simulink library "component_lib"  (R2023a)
settings: Solver=VariableStepAuto  StartTime=0.0  StopTime=10.0  RelTol=1e-3
undefined symbols (not defined in the file or in its folder): component_lib, ECCV_r, KoblenzTrier, mm, par, param_TD04, R1234yf_ph, SigIdentifier, Systems, TH0023_WP120, Thermal, V_nom
libraries: base_lib x166, $bdroot x164, simulink x2, slpidlib x1
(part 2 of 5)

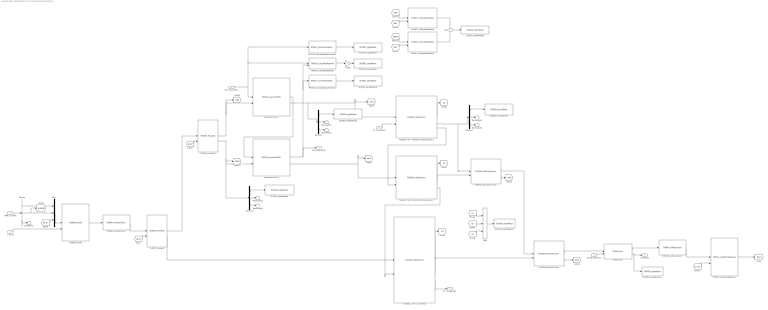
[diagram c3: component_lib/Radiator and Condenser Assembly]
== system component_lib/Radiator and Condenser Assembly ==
  AMB: (T,p,RH) : Inport
  v [m/s] : Inport  Port=2
  rel_fan_speed [-] : Inport  Port=3
  CL: (T1,p1,W1) : Inport  Port=4
  RF: (h1,p1,W1) : Inport  Port=5
  Add : Sum  Inputs=+++
  Condenser Pass 1 : $bdroot/Thermal Systems/RF0012_louverFinHEX  N_tub=40  T_L=0.95  T_p=10.15e-3  T_d=16e-3  N_ch=18  a=1.3e-3  b=0.58e-3  L_a=23  F_p=1.4e-3  L_p=1.7e-3  L_l=6.4e-3  H=8.15e-3  d_f=16e-3  F_d=16e-3  N_nod=5
  Condenser Pass 2 : $bdroot/Thermal Systems/RF0012_louverFinHEX  N_tub=40  T_L=0.95  T_p=10.15e-3  T_d=16e-3  N_ch=18  a=1.3e-3  b=0.58e-3  L_a=23  F_p=1.4e-3  L_p=1.7e-3  L_l=6.4e-3  H=8.15e-3  d_f=16e-3  F_d=16e-3  N_nod=5
  Demux{,1..3} (4 alike) : Demux  Outputs=3
  Gain2 : Gain  Gain=-1
  Mux : Mux  Inputs=3
  RF0013_calculateHeatflow : $bdroot/Thermal Systems/RF0013_calculateHeatflow
  RF0014_calculateVaporFraction : $bdroot/Thermal Systems/RF0014_calculateVaporFraction
  RF0014_calculateVaporFraction1 : $bdroot/Thermal Systems/RF0014_calculateVaporFraction
  Radiator core - behind condenser pass 1 : $bdroot/Thermal Systems/TH0002_radiatorCore  HtH=0.4060  StS=0.95  radmodel=52 mm
  Radiator core - behind condenser pass 2 : $bdroot/Thermal Systems/TH0002_radiatorCore  HtH=0.4060  StS=0.95  radmodel=52 mm
  Radiator core - uncovered : $bdroot/Thermal Systems/TH0002_radiatorCore  HtH=1.1- 2 * 0.4060  StS=0.95  radmodel=52 mm
  SC0002_signalRead1 : $bdroot/Data & Control/SC0002_signalRead  SigName=vaporFractionCondenserInlet
  SC0002_signalRead10 : $bdroot/Data & Control/SC0002_signalRead  SigName=vaporFractionCondenserOutlet
  SC0002_signalRead11 : $bdroot/Data & Control/SC0002_signalRead  SigName=fanPower
  SC0002_signalRead12 : $bdroot/Data & Control/SC0002_signalRead  SigName=radiatorCooling
  SC0002_signalRead2 : $bdroot/Data & Control/SC0002_signalRead  SigName=airTemperatureAfterCondenser
  SC0002_signalRead3 : $bdroot/Data & Control/SC0002_signalRead  SigName=airTemperatureAfterRadiator
  SC0002_signalRead4 : $bdroot/Data & Control/SC0002_signalRead  SigName=airTemperatureIntake
  SC0002_signalRead5 : $bdroot/Data & Control/SC0002_signalRead  SigName=condenserAirHeating
  SC0002_signalRead9 : $bdroot/Data & Control/SC0002_signalRead  SigName=condenserCooling
  Sum : Sum  Inputs=+|+
  TH0005_flowSplit : $bdroot/Thermal Systems/TH0005_flowSplit  SystemSampleTime=-1  VariantActivationTime=update diagram  Latency=0  AutoFrameSizeCalculation=off
  TH0005_flowSplit1 : $bdroot/Thermal Systems/TH0005_flowSplit  SystemSampleTime=-1  VariantActivationTime=update diagram  Latency=0  AutoFrameSizeCalculation=off
  TH0006_flowConfluence : $bdroot/Thermal Systems/TH0006_flowConfluence  gain=0.01
  TH0006_flowConfluence1 : $bdroot/Thermal Systems/TH0006_flowConfluence  gain=0.01
  TH0007_airRestriction : $bdroot/Thermal Systems/TH0007_airRestriction  A=0.8  zeta=0.3
  TH0007_airRestriction1 : $bdroot/Thermal Systems/TH0007_airRestriction  A=1  zeta=2.5
  TH0009_intake : $bdroot/Thermal Systems/TH0009_intake  zeta=0.9
  TH0010_fan : $bdroot/Thermal Systems/TH0010_fan  n_fan=4
  TH0011_outletFlowBalance : $bdroot/Thermal Systems/TH0011_outletFlowBalance  gain=0.05
  TH0017_calculateHeatflow : $bdroot/Thermal Systems/TH0017_calculateHeatflow
  TH0017_calculateHeatflow1 : $bdroot/Thermal Systems/TH0017_calculateHeatflow
  Terminator{,1..6} (7 alike) : Terminator
  P_fan [J/s] : Outport
  CL: (T2,p2,W2) : Outport  Port=2
  RF: (h2,p2,W2) : Outport  Port=3
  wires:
  Demux/2 -> Mux/2, [p_amb]
  Demux/1 -> Mux/1
  AMB: (T,p,RH)/1 -> Demux/1
  Radiator core - uncovered/3 -> CL: (T2,p2,W2)/1
  TH0010_fan/2 -> SC0002_signalRead11/1, P_fan [J/s]/1
  rel_fan_speed [-]/1 -> TH0010_fan/2
  v [m/s]/1 -> TH0009_intake/2
  TH0007_airRestriction/1 -> TH0005_flowSplit/1
  TH0007_airRestriction1/1 -> TH0011_outletFlowBalance/1
  TH0006_flowConfluence/1 -> TH0010_fan/1
  Mux/1 -> TH0009_intake/1
  TH0009_intake/1 -> TH0007_airRestriction/1
  Radiator core - uncovered/2 -> TH0006_flowConfluence/2
  [p_amb] -> TH0011_outletFlowBalance/2
  TH0005_flowSplit/2 -> Radiator core - uncovered/1
  TH0010_fan/1 -> TH0007_airRestriction1/1
  TH0011_outletFlowBalance/1 -> [W_in]
  [W_in] -> Mux/3
  Demux/3 -> Terminator/1
  CL: (T1,p1,W1)/1 -> Radiator core - behind condenser pass 1/2
  TH0005_flowSplit/1 -> TH0005_flowSplit1/1
  Condenser Pass 2/1 -> RF0013_calculateHeatflow/2, RF0014_calculateVaporFraction/1, RF: (h2,p2,W2)/1
  Condenser Pass 1/1 -> Condenser Pass 2/1
  Condenser Pass 1/2 -> [AIR1], Radiator core - behind condenser pass 1/1, Demux1/1
  Condenser Pass 2/2 -> [AIR2], Radiator core - behind condenser pass 2/1
  TH0005_flowSplit1/1 -> [AIR0], Condenser Pass 1/2
  Radiator core - behind condenser pass 1/3 -> Radiator core - behind condenser pass 2/2
  Radiator core - behind condenser pass 2/3 -> Radiator core - uncovered/2
  Radiator core - behind condenser pass 2/2 -> TH0006_flowConfluence1/2
  TH0006_flowConfluence1/1 -> TH0006_flowConfluence/1
  [split1] -> TH0005_flowSplit/2
  TH0006_flowConfluence/2 -> [split1]
  [split2] -> TH0005_flowSplit1/2
  TH0006_flowConfluence1/2 -> [split2]
  RF0013_calculateHeatflow/1 -> Gain2/1
  Gain2/1 -> SC0002_signalRead9/1
  Add/1 -> SC0002_signalRead12/1
  RF0014_calculateVaporFraction/1 -> SC0002_signalRead10/1
  RF0014_calculateVaporFraction1/1 -> SC0002_signalRead1/1
  RF: (h1,p1,W1)/1 -> RF0014_calculateVaporFraction1/1, RF0013_calculateHeatflow/1, Condenser Pass 1/1
  Radiator core - behind condenser pass 1/1 -> [Q1]
  Radiator core - behind condenser pass 2/1 -> [Q2]
  Radiator core - uncovered/1 -> [Q3]
  [Q1] -> Add/1
  [Q2] -> Add/2
  [Q3] -> Add/3
  Demux1/2 -> Terminator1/1
  Demux1/3 -> Terminator2/1
  Demux1/1 -> SC0002_signalRead2/1
  Radiator core - behind condenser pass 1/2 -> TH0006_flowConfluence1/1, Demux2/1
  Demux2/3 -> Terminator4/1
  Demux2/2 -> Terminator3/1
  Demux2/1 -> SC0002_signalRead3/1
  TH0005_flowSplit1/2 -> Demux3/1, Condenser Pass 2/2, [AIR00]
  Demux3/3 -> Terminator6/1
  Demux3/2 -> Terminator5/1
  Demux3/1 -> SC0002_signalRead4/1
  [AIR0] -> TH0017_calculateHeatflow/1
  [AIR1] -> TH0017_calculateHeatflow/2
  [AIR2] -> TH0017_calculateHeatflow1/2
  TH0017_calculateHeatflow/1 -> Sum/1
  TH0017_calculateHeatflow1/1 -> Sum/2
  Sum/1 -> SC0002_signalRead5/1
  [AIR00] -> TH0017_calculateHeatflow1/1

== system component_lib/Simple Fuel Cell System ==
  I [A] : Inport
  T [K] : Inport  Port=2
  Constant : Constant  Value=2.5e5
  Constant1 : Constant  Value=0.8
  Constant2 : Constant  Value=2.5e5
  Constant3 : Constant  Value=0.8
  Constant4 : Constant  Value=n
  EL0007_pukrushpan2004 : $bdroot/Electrochemistry/EL0007_pukrushpan2004  U_0=1  j_0=1e-3  alpha=0.25  ASR=1e-1  A_fc=420
  F0010_vaporSaturationPressure.m : base_lib/F0010_gasFlow/F0010_vaporSaturationPressure.m  SystemSampleTime=-1  VariantActivationTime=update diagram  Latency=0  AutoFrameSizeCalculation=off
  GE0002_dynHumidGasSupply : $bdroot/Gas Exchange/GE0002_dynHumidGasSupply  x_H2_dry=0  x_O2_dry=0.21
  GE0002_dynHumidGasSupply1 : $bdroot/Gas Exchange/GE0002_dynHumidGasSupply  x_H2_dry=1  x_O2_dry=0
  Gain : Gain  Gain=n_st
  Gain1 : Gain  Gain=n_st
  Gain2 : Gain  Gain=n_st
  Product{1..5} (5 alike) : Product
  SC0002_signalRead1 : $bdroot/Data & Control/SC0002_signalRead  SigName=fuelCellVoltage
  SC0002_signalRead3 : $bdroot/Data & Control/SC0002_signalRead  SigName=membraneWaterContent
  SC0002_signalRead4 : $bdroot/Data & Control/SC0002_signalRead  SigName=fuelCellPower
  SC0002_signalRead5 : $bdroot/Data & Control/SC0002_signalRead  SigName=vaporSaturationPressure
  SC0002_signalRead6 : $bdroot/Data & Control/SC0002_signalRead  SigName=singleCellVoltage
  SC0002_signalRead8 : $bdroot/Data & Control/SC0002_signalRead  SigName=fuelCellCurrent
  Subsystem1 : Subsystem
  V [V] : Outport
  Q_gen [J/s] : Outport  Port=2
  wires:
  Product1/1 -> Gain1/1
  Product2/1 -> [W_an], Gain/1
  Product5/1 -> [W_ca]
  Constant4/1 -> Product1/2, Product2/2, Product5/2, Product3/2
  EL0007_pukrushpan2004/3 -> Product5/1
  EL0007_pukrushpan2004/2 -> Product2/1
  EL0007_pukrushpan2004/5 -> Product3/1
  Product4/1 -> SC0002_signalRead4/1
  EL0007_pukrushpan2004/4 -> SC0002_signalRead3/1
  T [K]/1 -> F0010_vaporSaturationPressure.m/1, EL0007_pukrushpan2004/4, EL0007_pukrushpan2004/5, EL0007_pukrushpan2004/6, GE0002_dynHumidGasSupply1/1, GE0002_dynHumidGasSupply/1
  F0010_vaporSaturationPressure.m/1 -> SC0002_signalRead5/1
  Gain/1 -> Subsystem1/1(In1)
  Gain1/1 -> V [V]/1, SC0002_signalRead1/1, Product4/2
  Product3/1 -> Gain2/1
  Gain2/1 -> Q_gen [J/s]/1
  GE0002_dynHumidGasSupply1/1 -> EL0007_pukrushpan2004/2
  GE0002_dynHumidGasSupply/1 -> EL0007_pukrushpan2004/3
  I [A]/1 -> EL0007_pukrushpan2004/1, SC0002_signalRead8/1, Product4/1
  EL0007_pukrushpan2004/1 -> SC0002_signalRead6/1, Product1/1
  Constant/1 -> GE0002_dynHumidGasSupply/2
  Constant1/1 -> GE0002_dynHumidGasSupply/3
  Constant3/1 -> GE0002_dynHumidGasSupply1/3
  Constant2/1 -> GE0002_dynHumidGasSupply1/2

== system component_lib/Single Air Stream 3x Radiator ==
  AMB: (T,p,RH) : Inport
  v [m/s] : Inport  Port=2
  rel_fan_speed [-] : Inport  Port=3
  CL A: (T1,p1,W1) : Inport  Port=4
  CL B: (T1,p1,W1) : Inport  Port=5
  CL C: (T1,p1,W1) : Inport  Port=6
  Battery Circuit Radiator : $bdroot/Thermal Systems/TH0002_radiatorCore  HtH=1.1  StS=0.95  radmodel=52 mm
  Demux : Demux  Outputs=3
  Fuel Cell Circuit Radiator : $bdroot/Thermal Systems/TH0002_radiatorCore  HtH=1.1  StS=0.95  radmodel=52 mm
  Fuel Cell Circuit Radiator1 : $bdroot/Thermal Systems/TH0002_radiatorCore  HtH=1.1  StS=0.95  radmodel=52 mm
  Mux : Mux  Inputs=3
  TH0003_coolantTank{,1..5} (6 alike) : $bdroot/Thermal Systems/TH0003_coolantTank  StS=0.95  D_con=0.055  T_0=286  radmodel=52 mm
  TH0004_radiatorPlugFlow : $bdroot/Thermal Systems/TH0004_radiatorPlugFlow  HtH=1.1  StS=0.95  T_0=286  radmodel=52 mm
  TH0004_radiatorPlugFlow1 : $bdroot/Thermal Systems/TH0004_radiatorPlugFlow  HtH=1.1  StS=0.95  T_0=286  radmodel=52 mm
  TH0004_radiatorPlugFlow2 : $bdroot/Thermal Systems/TH0004_radiatorPlugFlow  HtH=1.1  StS=0.95  T_0=286  radmodel=52 mm
  TH0007_airRestriction : $bdroot/Thermal Systems/TH0007_airRestriction  A=0.8  zeta=0.3
  TH0007_airRestriction1 : $bdroot/Thermal Systems/TH0007_airRestriction  A=1  zeta=2.5
  TH0009_intake : $bdroot/Thermal Systems/TH0009_intake  zeta=0.9
  TH0010_fan : $bdroot/Thermal Systems/TH0010_fan  n_fan=10
  TH0011_outletFlowBalance : $bdroot/Thermal Systems/TH0011_outletFlowBalance  gain=0.05
  P_fan [J/s] : Outport
  CL A: (T2,p2,W2) : Outport  Port=2
  CL B: (T2,p2,W2) : Outport  Port=3
  CL C: (T2,p2,W2) : Outport  Port=4
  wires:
  Demux/2 -> Mux/2, [p_amb]
  Demux/1 -> Mux/1
  AMB: (T,p,RH)/1 -> Demux/1
  TH0003_coolantTank1/1 -> CL A: (T2,p2,W2)/1
  TH0010_fan/2 -> P_fan [J/s]/1
  rel_fan_speed [-]/1 -> TH0010_fan/2
  v [m/s]/1 -> TH0009_intake/2
  TH0004_radiatorPlugFlow/1 -> TH0003_coolantTank1/1
  TH0007_airRestriction1/1 -> TH0011_outletFlowBalance/1
  CL A: (T1,p1,W1)/1 -> TH0003_coolantTank/1
  Mux/1 -> TH0009_intake/1
  TH0009_intake/1 -> TH0007_airRestriction/1
  TH0003_coolantTank/1 -> Battery Circuit Radiator/2
  [p_amb] -> TH0011_outletFlowBalance/2
  TH0007_airRestriction/1 -> Battery Circuit Radiator/1
  TH0010_fan/1 -> TH0007_airRestriction1/1
  Battery Circuit Radiator/3 -> TH0004_radiatorPlugFlow/1
  TH0011_outletFlowBalance/1 -> [W_in]
  [W_in] -> Mux/3
  Battery Circuit Radiator/2 -> Fuel Cell Circuit Radiator/1
  Fuel Cell Circuit Radiator/2 -> Fuel Cell Circuit Radiator1/1
  TH0004_radiatorPlugFlow1/1 -> TH0003_coolantTank2/1
  TH0003_coolantTank2/1 -> CL B: (T2,p2,W2)/1
  Fuel Cell Circuit Radiator/3 -> TH0004_radiatorPlugFlow1/1
  Fuel Cell Circuit Radiator1/3 -> TH0004_radiatorPlugFlow2/1
  TH0003_coolantTank3/1 -> CL C: (T2,p2,W2)/1
  TH0004_radiatorPlugFlow2/1 -> TH0003_coolantTank3/1
  TH0003_coolantTank4/1 -> Fuel Cell Circuit Radiator/2
  CL B: (T1,p1,W1)/1 -> TH0003_coolantTank4/1
  TH0003_coolantTank5/1 -> Fuel Cell Circuit Radiator1/2
  CL C: (T1,p1,W1)/1 -> TH0003_coolantTank5/1
  Fuel Cell Circuit Radiator1/2 -> TH0010_fan/1

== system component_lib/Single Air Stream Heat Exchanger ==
  AMB: (T,p,RH) : Inport
  v [m/s] : Inport  Port=2
  rel_fan_speed [-] : Inport  Port=3
  CL: (T1,p1,W1) : Inport  Port=4
  Demux : Demux  Outputs=3
  Mux : Mux  Inputs=3
  Radiator core - exposed : $bdroot/Thermal Systems/TH0002_radiatorCore  HtH=0.6  StS=0.6  radmodel=52 mm
  TH0003_coolantTank : $bdroot/Thermal Systems/TH0003_coolantTank  StS=0.95  D_con=0.055  T_0=286  radmodel=52 mm
  TH0003_coolantTank1 : $bdroot/Thermal Systems/TH0003_coolantTank  StS=0.95  D_con=0.055  T_0=286  radmodel=52 mm
  TH0004_radiatorPlugFlow : $bdroot/Thermal Systems/TH0004_radiatorPlugFlow  HtH=1.1  StS=0.95  T_0=286  radmodel=52 mm
  TH0007_airRestriction : $bdroot/Thermal Systems/TH0007_airRestriction  A=0.8  zeta=0.3
  TH0007_airRestriction1 : $bdroot/Thermal Systems/TH0007_airRestriction  A=1  zeta=2.5
  TH0009_intake : $bdroot/Thermal Systems/TH0009_intake  zeta=0.9
  TH0010_fan : $bdroot/Thermal Systems/TH0010_fan  n_fan=4
  TH0011_outletFlowBalance : $bdroot/Thermal Systems/TH0011_outletFlowBalance  gain=0.05
  P_fan [J/s] : Outport
  CL: (T2,p2,W2) : Outport  Port=2
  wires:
  Demux/2 -> Mux/2, [p_amb]
  Demux/1 -> Mux/1
  AMB: (T,p,RH)/1 -> Demux/1
  TH0003_coolantTank1/1 -> CL: (T2,p2,W2)/1
  TH0010_fan/2 -> P_fan [J/s]/1
  rel_fan_speed [-]/1 -> TH0010_fan/2
  v [m/s]/1 -> TH0009_intake/2
  TH0004_radiatorPlugFlow/1 -> TH0003_coolantTank1/1
  TH0007_airRestriction1/1 -> TH0011_outletFlowBalance/1
  CL: (T1,p1,W1)/1 -> TH0003_coolantTank/1
  Mux/1 -> TH0009_intake/1
  TH0009_intake/1 -> TH0007_airRestriction/1
  TH0003_coolantTank/1 -> Radiator core - exposed/2
  [p_amb] -> TH0011_outletFlowBalance/2
  TH0007_airRestriction/1 -> Radiator core - exposed/1
  TH0010_fan/1 -> TH0007_airRestriction1/1
  Radiator core - exposed/3 -> TH0004_radiatorPlugFlow/1
  TH0011_outletFlowBalance/1 -> [W_in]
  [W_in] -> Mux/3
  Radiator core - exposed/2 -> TH0010_fan/1

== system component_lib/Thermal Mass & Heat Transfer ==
  Q_in [J/s] : Inport
  CL: (T1,p1,W1) : Inport  Port=2
  Sum : Sum  Inputs=|+-
  TH0011_coolingChannel : $bdroot/Thermal Systems/TH0011_coolingChannel  d=d  L=L  n_ch=n
  TH0011_thermalMass : $bdroot/Thermal Systems/TH0011_thermalMass  m=m  cp=cp  T_0=T_0
  T_ [K] : Outport
  CL: (T2,p2,W2) : Outport  Port=2
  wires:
  Sum/1 -> TH0011_thermalMass/1
  TH0011_thermalMass/1 -> T_ [K]/1, TH0011_coolingChannel/1
  TH0011_coolingChannel/1 -> Sum/2
  Q_in [J/s]/1 -> Sum/1
  CL: (T1,p1,W1)/1 -> TH0011_coolingChannel/2
  TH0011_coolingChannel/2 -> CL: (T2,p2,W2)/1

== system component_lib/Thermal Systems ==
  note: TitanX Radiator blockset
  RF0003_compressor : Subsystem  mask{V_disp=0.00017, N_ref=2000}
      mask prompts: V_disp "Displacement Volume [m3]:"; N_ref "Refrence Speed [rpm]:"
      mask init:
      | % fluid properties
      | 
      | par = struct;
      | par.V_disp = V_disp;
      | par.N_ref  = N_ref;
      | 
      | setRefrigerantProperties;
  RF0004_smoothTube : Subsystem  mask{D=8e-3, L=1}
      mask prompts: D "Tube diameter [m]:"; L "Tube length [m]:"
      mask init:
      | % fluid properties
      | 
      | par = struct;
      | par.D = D;
      | par.L = L;
      | 
      | setRefrigerantProperties;
  RF0005_expansionValve : Subsystem  mask{D=1.8e-3, p_min=150e3}
      mask prompts: D "Orifice diameter [m]:"; p_min "Minimum Downstream Pressure [Pa]:"
      mask init:
      | % fluid properties
      | 
      | setRefrigerantProperties;
      | 
      | par.D = D;
  RF0007_PHEX : Subsystem  mask{N_ch=10, L=180e-3, B=65e-3, H=2e-3, t=0.3e-3, D_h=2.61e-3, N_nod=10}
      mask prompts: N_ch "Plates [-]:"; L "Length [m]:"; B "Width [m]:"; H "Height [m]:"; t "Plate thickness [m]"; D_h "Hydraulic Diameter [m]:"; N_nod "Nodes [even integer]"
      mask init:
      | % fluid properties
      | 
      | setRefrigerantProperties;
      | setCoolantProperties;
      | 
      | % Linearly spaced nodes
      | dx = L ./ N_nod;
      | 
      | % flow cross section area
      | A_c = H .* B;
      | 
      | % Volume per node
      | V = B .* H .* dx;
      | 
      | % aluminium properties
      | cp_w     = 0.9e3; % [J/kg K] specific heat
      | k_w      = 237;   % [W / mK] thermal conductivity
      | rho_w    = 2710;
      | A_w      = t .* B;
      | V_w      = t .* B .* dx;
      | d_w      = dx;
      | 
      | % hydraulic diameter
      | par.D_h = D_h;
      | 
      | % heat transfer area for each node
      | A =  2 .* B .* dx;
  RF0008_receiver : Subsystem  mask{V=1e-3, h0=280e3, p0=1e6, p_gain=1e3}
      mask prompts: V "Volume [m3]:"; h0 "Enthalpy [J/kg]:"; p0 "Pressure [Pa]:"; p_gain "Pressure gain:"
      mask init:
      | % fluid properties
      | par = struct;
      | setRefrigerantProperties;
  RF0010_calculateSuperHeat : Subsystem
      mask init:
      | % fluid properties
      | par = struct;
      | setRefrigerantProperties;
  RF0011_calculateSubCool : Subsystem
      mask init:
      | % fluid properties
      | par = struct;
      | setRefrigerantProperties;
  RF0012_louverFinHEX : Subsystem  mask{N_tub=30, T_L=0.3, T_p=10.15e-3, T_d=16e-3, N_ch=18, a=1.3e-3, b=0.58e-3, L_a=23, F_p=1.4e-3, L_p=1.7e-3, L_l=6.4e-3, H=8.15e-3, d_f=16e-3, F_d=16e-3, N_nod=10}
      mask prompts: N_tub "Nr. of Tubes [-]"; T_L "Tube length [m]:"; T_p "Tube pitch [m]:"; T_d "Tube depth [m]:"; N_ch "Minichannels per tube [-]"; a "Minichannel height [m]"; b "Minichannel width [m]"; L_a "Louver angle [deg]:"; F_p "Fin Pitch [m]:"; L_p "Louver Pitch [m]:"; L_l "Louver length [m]:"; H "Fin height [m]:"; d_f "Fin thickness [m]:"; F_d "Flow depth [m]:"; N_nod "Nodes [even integer]"
      mask init:
      | % fluid properties
      | 
      | setRefrigerantProperties;
      | setCoolantProperties;
      | setAirProperties;
      | 
      | % channel parameters
      | par.a = a;
      | par.b = b;
      | 
      | % Louver fin parameters
      | par.L_a  = L_a;  % Louver angle [deg]
      | par.F_p  = F_p;  % Fin pitch [m]
      | par.L_p  = L_p;  % Louver pitch [m]
      | par.L_l  = L_l;  % Louver length [m]
      | par.H    = H;    % Fin height [m]
      | par.T_p  = T_p;  % Tube pitch [m]
      | par.T_d  = T_d;  % Tube depth [m]
      | par.d_f  = d_f;  % Fin thickness [m]
      | par.F_d  = F_d;  % Flow depth [m]
      | 
      | % Aluminium properties
      | cp_w  = 0.9e3; % [J/kg K] specific heat
      | k_w   = 237;   % [W / mK] thermal conductivity
      | rho_w = 2710;
      | 
      | par.cp_w = cp_w;
      | par.k_w = k_w;
      | par.rho_w = rho_w;
      | 
      | 
      | % uniformly spaced nodes
      | dx = T_L ./ N_nod;
      | 
      | % Inner channel surface
      | A_wr = 2.*(a+b) .* dx .*  N_ch;
      | 
      | % Hydraulic diameter
      | D_h =  2 .* a .* b /(a + b);
      | par.D_h = D_h;
      | 
      | % Channel volume per node
      | V = N_ch .* a .* b .* dx;
      | 
      | % approximate number of fins between two tubes
      | n_fin = T_L./F_p;
      | 
      | % Fin surface area per node per tube
      | A_f =  L_l .* F_d .* n_fin ./ N_nod;
      | par.A_f = A_f;
      | 
      | % Tube surfae area per node
      | A_tub = 2 .* dx .* T_d;
      | 
      | % Total surface area per node
      | A_o = A_f + A_tub;
      | par.A_o = A_o;
      | 
      | % free flow cross section area per tube
      | A_fr = T_p .*  T_L;
      | 
      | % minimum cross section area per tube
      | A_min = H .* T_L  - atan( L_a * pi / 180 ) * L_p .* L_l;
      | 
      | % contraction ratio
      | par.sigma = A_fr ./ A_min;
      | 
      | % metal volume per node
      | V_w = (T_d .* (T_p - H)  - a.*b*N_ch ) * dx + A_f .* d_f; 
      | 
      | % node distance
      | d_w = dx;
      | A_w = (T_d .* (T_p - H)  - a.*b*N_ch );
      | 
      | % air volume per node
      | V_air = A_min .* F_d ./ N_nod;
  RF0013_calculateHeatflow : Subsystem
      mask init:
      | % fluid properties
      | par = struct;
      | setRefrigerantProperties;
      | setCoolantProperties;
  RF0014_calculateVaporFraction : Subsystem
      mask init:
      | % fluid properties
      | par = struct;
      | setRefrigerantProperties;
  RF0015_controlVolume : Subsystem  mask{V=1e-3, p0=200e3, h0=420e3}
      mask prompts: V "Volume [m3]"; p0 "Pressure [Pa]:"; h0 "Enthalpy [J/kg]:"
      mask init:
      | % fluid properties
      | par = struct;
      | setRefrigerantProperties;
  RF0016_split : Subsystem
      mask init:
      | % fluid properties
      | 
      | 
      | setRefrigerantProperties;
  RF0017_merge : Subsystem  mask{V=1e-3}
      mask prompts: V "Volume [m3]:"
      mask init:
      | % fluid properties
      | 
      | 
      | setRefrigerantProperties;
  RF0018_calculateTemperature : Subsystem
      mask init:
      | % fluid properties
      | par = struct;
      | setRefrigerantProperties;
  TH0002_radiatorCore : Subsystem  mask{HtH=1.1, StS=0.95, radmodel=52 mm}
      mask prompts: HtH "Effective header to header [m]:"; StS "Effective sideplate to sideplate [m]:"; radmodel "Core depth [m]:"
      mask init:
      | % parameter struct
      | par = struct;
      | 
      | % % get parameters
      | % par.HtH = eval(get_param(gcb, 'HtH'));
      | % par.StS = eval(get_param(gcb, 'StS'));
      | 
      | par.HtH = HtH;
      | par.StS = StS;
      | 
      | % Geometry
      | par.A_face = HtH * StS;
      | 
      | % Total heat transfer coefficient model:
      | par.cUexp = [0.7; 0.8];
      | 
      | switch radmodel
      |     
      |         case '19 mm'
      |         % Core depth
      |         par.CdT = 24e-3;
      |         
      |         % Heat trf. coefficient coefficients
      |         par.cU = [1.118075425066717e-04;
      |                   5.580064095289469e-04;
      |                   2.895685646303412e-05];
      |         
      |         % pressure drop coefficients
      |         par.c_dp_air = [37.253944105671480;
      |                          2.916659649936296e+02];         
      |         par.c_dp_clt = [19.727883408911566;
      |                          5.313528394369467];
      |         
      |         % relative area factors:
      |         rel_air = 0.752767994911226;
      |         rel_clt = 0.127946647958308;
      |     
      |     
      |         case '24 mm'
      |         % Core depth
      |         par.CdT = 24e-3;
      |         
      |         % Heat trf. coefficient coefficients
      |         par.cU = [9.815616404383520e-05;
      |                   4.676700861536502e-04;
      |                   2.415838699598361e-05];
      |         
      |         % pressure drop coefficients
      |         par.c_dp_air = [45.764851256613420;
      |                          2.404056250729179e+02];         
      |         par.c_dp_clt = [18.543378283094310;
      |                          5.151503273505832];
      |         
      |         % relative area factors:
      |         rel_air = 0.733387923444172;
      |         rel_clt = 0.132407142901122;
      |     
      |     
      |     
      |     case '42 mm'
      |         % Core depth
      |         par.CdT = 42e-3;
      |         
      |         % Heat trf. coefficient coefficients
      |         par.cU = [5.544027785616380e-05; 
      |                   2.449228920498670e-04; 
      |                   1.520415888705416e-05];
      |         
      |         % pressure drop coefficients
      |         par.c_dp_air = [36.973761781463810;
      |                          2.758340137219987e+02];
      |         par.c_dp_clt = [19.845956523612838;
      |                          5.112131585795914];
      |         
      |         % relative area factors:
      |         rel_air = 0.752767994911226;
      |         rel_clt = 0.115761252914660;
      |         
      |     case '52 mm'
      |         % Core depth
      |         par.CdT = 52e-3;
      |         
      |         % Heat trf. coefficient coefficients
      |         par.cU = [5.19516413772077e-05;
      |                   0.000198353781023090;
      |                   1.28249375163373e-05];
      |         
      |         % pressure drop coefficients
      |         par.c_dp_air = [46.462548129557995;
      |                          2.255631867184913e+02];
      |         par.c_dp_clt = [18.741626674634468;
      |                          4.871890188700768];
      |         
      |         % relative area factors:
      |         rel_air = 0.7334;
      |         rel_clt = 0.1222;
      | end
      | 
      | 
      | % Flow areas:
      | par.A_air  = rel_air * par.A_face; % Characteristic flow area
      | par.A_clt  = rel_clt * par.CdT * StS;  % Characteristic flow area
      | 
      | % fluid properties
      | setCoolantProperties;
      | setAirProperties;
  TH0003_coolantTank : Subsystem  mask{StS=0.95, D_con=0.055, T_0=273 + 25, radmodel=52 mm}
      mask prompts: StS "Sideplate to sideplate [m]"; D_con "Connector internal diameter [m]:"; T_0 "Temperature initial condition [K]:"; radmodel "Core depth [mm]:"
      mask init:
      | par = struct;
      | 
      | % fluid properties
      | setCoolantProperties;
      | setAirProperties;
      | 
      | % pressure drop coeffcient
      | par.zeta = 3;
      | 
      | % set core depth
      | switch radmodel
      |     
      |     case '19 mm'
      |         % Core depth
      |         par.CdT = 19e-3;
      |         
      |     case '24 mm'
      |         % Core depth
      |         par.CdT = 24e-3;
      |     
      |     case '42 mm'
      |         % Core depth
      |         par.CdT = 42e-3;
      |         
      |     case '52 mm'
      |         % Core depth
      |         par.CdT = 52e-3;
      | end
      | 
      | % Geometry
      | % tank volume
      | par.V = par.CdT.^2 * StS;
      | 
      | % inlet area
      | par.A_con = D_con.^2 .* pi/4;
  TH0004_radiatorPlugFlow : Subsystem  mask{HtH=1.1, StS=0.95, T_0=286, radmodel=52 mm}
      mask prompts: HtH "Header to header [m]:"; StS "Sideplate to sideplate [m]:"; T_0 "Temperature initial condition [K]:"; radmodel "Core depth [mm]:"
      mask init:
      | par = struct;
      | 
      | % get parameters
      | % par.HtH = eval(get_param(gcb, 'HtH'));
      | % par.StS = eval(get_param(gcb, 'StS'));
      | 
      | par.HtH = HtH;
      | par.StS = StS;
      | 
      | % fluid properties
      | setCoolantProperties;
      | setAirProperties;
      | 
      | 
      | % set core depth
      | switch radmodel
      |     case '42 mm'
      |         % Core depth
      |         par.CdT = 42e-3;
      |         
      |     case '52 mm'
      |         % Core depth
      |         par.CdT = 52e-3;
      | end
  TH0005_flowSplit : Subsystem
      mask init:
      | % fluid properties
      | setCoolantProperties;
      | setAirProperties;
  TH0006_flowConfluence : Subsystem  mask{gain=0.01}
      mask prompts: gain "Flow balance gain [-]:"
      mask init:
      | % fluid properties
      | setCoolantProperties;
      | setAirProperties;
  TH0007_airRestriction : Subsystem  mask{A=0.8, zeta=0.3}
      mask prompts: A "Area [m2]:"; zeta "Pressure drop coefficient [-]:"
      mask init:
      | % get parameters
      | % par.A    = eval(get_param(gcb, 'A'));
      | % par.zeta = eval(get_param(gcb, 'zeta'));
      | 
      | par.A    = A;
      | par.zeta = zeta;
      | 
      | % fluid properties
      | setCoolantProperties;
      | setAirProperties;
  TH0008_condenser : Subsystem  mask{HtH=0.85, StS=0.35, cdsmodel=16 mm}
      mask prompts: HtH "Header to header [m]:"; StS "Sideplate to sideplate [m]:"; cdsmodel "Core depth [m]:"
      mask init:
      | % parameter struct
      | par = struct;
      | 
      | % get parameters
      | % par.HtH = eval(get_param(gcb, 'HtH'));
      | % par.StS = eval(get_param(gcb, 'StS'));
      | 
      | par.HtH = HtH;
      | par.StS = StS;
      | 
      | 
      | switch cdsmodel
      |     case '16 mm'
      |         % Core depth
      |         par.CdT = 16-3;
      |         
      |         % pressure drop coefficients
      |         par.c_dp = [2.5; 6];
      |         
      |         
      |     case '18.8 mm'
      |         % Core depth
      |         par.CdT = 18.8e-3;
      |         
      |         % pressure drop coefficients
      |         par.c_dp = [2.7; 11];
      | end
      | 
      | % fluid properties
      | setCoolantProperties;
      | setAirProperties;
  TH0009_intake : Subsystem  mask{zeta=0.9}
      mask prompts: zeta "Pressure increase coefficient [-]:"
      mask init:
      | % get parameters
      | % par.zeta = eval(get_param(gcb, 'zeta'));
      | par.zeta = zeta;
      | 
      | % fluid properties
      | setCoolantProperties;
      | setAirProperties;
  TH0010_fan : Subsystem  mask{n_fan=4}
      mask prompts: n_fan "Nr. of fans [-]:"
      mask init:
      | % parameter struct
      | par = struct;
      | 
      | % get parameters
      | % par.n_fan = eval(get_param(gcb, 'n_fan'));
      | par.n_fan = n_fan;
      | 
      | 
      | % fan parameters
      | par.dpr   = -200;
      | par.q0    = 4290/3600;
      | par.dp0   = 800;
      | par.P_nom = 832;
      | 
      | 
      | % fluid properties
      | setCoolantProperties;
      | setAirProperties;
  TH0011_coolingChannel : Subsystem  mask{d=2e-3, L=50e-2, n_ch=1, e=0.006e-3}
      mask prompts: d "Hydraulic diameter [m]:"; L "Length [m]:"; n_ch "Nr. of channels [-]:"; e "Roughness [-]:"
      mask init:
      | % parameter struct
      | par = struct;
      | par.d = d;
      | par.L = L;
      | par.e = e;
      | 
      | % fluid properties
      | setCoolantProperties;
      | setAirProperties;
  TH0011_outletFlowBalance : Subsystem  mask{gain=0.05}
      mask prompts: gain "Dyn. balancing factor [m]:"
      mask init:
      | % fluid properties
      | setCoolantProperties;
      | setAirProperties;
  TH0011_pipe : Subsystem  mask{d=5e-2, L=1, e=0.006e-3, T_0=273 + 20}
      mask prompts: d "Diameter [m]:"; L "Length [m]:"; e "Roughness [m]:"; T_0 "Initial temperature [K]:"
      mask init:
      | % parameter struct
      | par = struct;
      | 
      | % get parameters
      | % par.d = eval(get_param(gcb, 'd'));
      | % par.L = eval(get_param(gcb, 'L'));
      | 
      | par.d = d;
      | par.L = L;
      | par.e = e;
      | 
      | % fluid properties
      | setCoolantProperties;
      | setAirProperties;
  TH0011_thermalMass : Subsystem  mask{m=34, cp=691, T_0=273 + 20}
      mask prompts: m "Mass [kg]:"; cp "Heat capacity [J/kgK]:"; T_0 "Initial temperature [K]:"
      mask init:
      | % fluid properties
      | setCoolantProperties;
      | setAirProperties;
  TH0012_equalSplitMerge : Subsystem  mask{n=1}
      mask prompts: n "Split/merge flow [-]"
      mask init:
      | % fluid properties
      | setCoolantProperties;
      | setAirProperties;
  TH0013_tank : Subsystem  mask{V=5e-3, T0=273.15 + 80}
      mask prompts: V "Volume [m3]:"; T0 "Temperature [K]:"
      mask init:
      | % fluid properties
      | setCoolantProperties;
      | setAirProperties;
  TH0014_valve : Subsystem  mask{d=10e-2, dr=5e-2, C_d=0.9}
      mask prompts: d "Inlet port diameter [m]:"; dr "Restriction diameter [m]:"; C_d "Discharge coefficient [-]:"
      mask init:
      | % parameter struct
      | par = struct;
      | 
      | % get parameters
      | % par.d    = eval(get_param(gcb, 'd'));
      | % par.dr   = eval(get_param(gcb, 'dr'));
      | % par.C_d  = eval(get_param(gcb, 'C_d'));
      | 
      | par.d    = d;
      | par.dr   = dr;
      | par.C_d  = C_d;
      | 
      | 
      | % fluid properties
      | setCoolantProperties;
      | setAirProperties;
  TH0015_totalHeatTransfer : Subsystem  mask{T_max=273+100, T_min=273}
      mask prompts: T_max "Max. Temperature [K]:"; T_min "Min.Temperature [K]"
      mask init:
      | % parameter struct
      | par = struct;
      | 
      | % fluid properties
      | setCoolantProperties;
      | setAirProperties;
  TH0016_calculateHeatflow : Subsystem
      mask init:
      | % fluid properties
      | par = struct;
      | setRefrigerantProperties;
      | setCoolantProperties;
  TH0017_calculateHeatflow : Subsystem
      mask init:
      | % fluid properties
      | par = struct;
      | setRefrigerantProperties;
      | setCoolantProperties;
      | setAirProperties;
  TH0018_PHEX : Subsystem  mask{N_ch=10, L=180e-3, B=65e-3, H=2e-3, t=0.3e-3, D_h=2.61e-3, N_nod=10}
      mask prompts: N_ch "Plates [-]:"; L "Length [m]:"; B "Width [m]:"; H "Height [m]:"; t "Plate thickness [m]"; D_h "Hydraulic Diameter [m]:"; N_nod "Nodes [even integer]"
      mask init:
      | % fluid properties
      | 
      | setRefrigerantProperties;
      | setCoolantProperties;
      | 
      | % Linearly spaced nodes
      | dx = L ./ N_nod;
      | 
      | % flow cross section area
      | A_c = H .* B;
      | 
      | % Volume per node
      | V = B .* H .* dx;
      | 
      | % aluminium properties
      | cp_w     = 0.9e3; % [J/kg K] specific heat
      | k_w      = 237;   % [W / mK] thermal conductivity
      | rho_w    = 2710;
      | A_w      = t .* B;
      | V_w      = t .* B .* dx;
      | d_w      = dx;
      | 
      | % hydraulic diameter
      | par.D_h = D_h;
      | 
      | % heat transfer area for each node
      | A =  2 .* B .* dx;
  TH0019_airTotalHeatTransfer : Subsystem
      mask init:
      | % parameter struct
      | par = struct;
      | 
      | % fluid properties
      | setCoolantProperties;
      | setAirProperties;
  TH0020_cm100hp : Subsystem
      mask init:
      | % parameter struct
      | par   = struct;
      | 
      | % fluid properties
      | setCoolantProperties;
      | setAirProperties;
  TH0020_staticPressureDrop : Subsystem  mask{dp=1e4}
      mask prompts: dp "Pressure drop [Pa]:"
      mask init:
      | % parameter struct
      | par = struct;
      | 
      | % fluid properties
      | setCoolantProperties;
      | setAirProperties;
  TH0021_tank : Subsystem  mask{V=5e-3, T0=273.15 + 80}
      mask prompts: V "Volume [m3]:"; T0 "Temperature [K]:"
      mask init:
      | % fluid properties
      | setCoolantProperties;
      | setAirProperties;
  TH0022_restriction : Subsystem  mask{d=3.5e-3, C=0.8}
      mask prompts: d "Diameter [m]:"; C "Discharge coef. [-]"
      mask init:
      | % parameter struct
      | par = struct;
      | 
      | % get parameters
      | % par.d = eval(get_param(gcb, 'd'));
      | % par.L = eval(get_param(gcb, 'L'));
      | 
      | par.d = d;
      | par.C = C;
      | 
      | % fluid properties
      | setCoolantProperties;
      | setAirProperties;
  TH0023_WP120 : Subsystem
      mask init:
      | % parameter struct
      | par   = struct;
      | 
      | % fluid properties
      | setCoolantProperties;
      | setAirProperties;
  TH0024_WP150 : Subsystem  AncestorBlock=component_lib/Thermal Systems/TH0023_WP120
      mask init:
      | % parameter struct
      | par   = struct;
      | 
      | % fluid properties
      | setCoolantProperties;
      | setAirProperties;

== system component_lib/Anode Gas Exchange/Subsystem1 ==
  W_an : Inport
  W_an_reacted : Inport  Port=2
  Demux : Demux
  Demux1 : Demux
  Divide : Product  Inputs=*/
  Gain : Gain  Gain=-1
  SC0002_signalRead11 : $bdroot/Data & Control/SC0002_signalRead  SigName=anodeStoichiometry
  Saturation : Saturate  UpperLimit=10  LowerLimit=-10
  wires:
  Divide/1 -> Saturation/1
  W_an/1 -> Demux/1
  Demux/1 -> Divide/1
  W_an_reacted/1 -> Gain/1
  Gain/1 -> Demux1/1
  Demux1/1 -> Divide/2
  Saturation/1 -> SC0002_signalRead11/1

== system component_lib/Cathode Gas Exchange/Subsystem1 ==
  W_ca : Inport
  W_ca_reacted : Inport  Port=2
  Demux : Demux
  Demux1 : Demux
  Divide : Product  Inputs=*/
  Gain : Gain  Gain=-1
  SC0002_signalRead11 : $bdroot/Data & Control/SC0002_signalRead  SigName=cathodeStoichiometry
  Saturation : Saturate  UpperLimit=10  LowerLimit=0
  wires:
  Divide/1 -> Saturation/1
  W_ca/1 -> Demux/1
  W_ca_reacted/1 -> Gain/1
  Gain/1 -> Demux1/1
  Saturation/1 -> SC0002_signalRead11/1
  Demux/2 -> Divide/1
  Demux1/2 -> Divide/2

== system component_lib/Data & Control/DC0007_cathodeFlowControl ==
  note: Oxygen flow [kg/s]
  note: Reference oxygen flow [kg/s]
  I_fc [A] : Inport
  W_ca [kg/s] : Inport  Port=2
  Cells in FC stack : Constant  Value=n_cell
  F0003_reactionFlow.m : base_lib/F0003_pukrushpan2004/F0003_reactionFlow.m  SystemSampleTime=-1  VariantActivationTime=update diagram  Latency=0  AutoFrameSizeCalculation=off
  Gain : Gain  Gain=1e5
  Gain1 : Gain  Gain=-1
  Oxygen mass fraction in dry air : Constant  Value=0.23
  Oxygen stoichiometry reference : Constant  Value=lambda_O2_ref
  PID Controller : slpidlib/PID Controller  Controller=PID  Form=Parallel  TimeDomain=Continuous-time  UseExternalTs=off  SampleTime=-1  IntegratorMethod=Forward Euler  FilterMethod=Forward Euler  ControllerParametersSource=internal  P=1  I=1  UseKiTs=off  D=0  N=100  UseFilter=on  TunerSelectOption=Transfer Function Based (PID Tuner App)  InitialConditionSource=internal  InitialConditionForIntegrator=0  InitialConditionForFilter=0  DifferentiatorICPrevScaledInput=0  ExternalReset=none  TrackingMode=off  Kt=1  LimitOutput=on  SatLimitsSource=internal  UpperSaturationLimit=2e4  LowerSaturationLimit=3e3  LinearizeAsGain=on  AntiWindupMode=back-calculation  Kb=1e-1  LimitIntegrator=off  UpperIntegratorSaturationLimit=inf  LowerIntegratorSaturationLimit=-inf  POutMin=[]  POutMax=[]  IOutMin=[]  IOutMax=[]  DOutMin=[]  DOutMax=[]  NOutMin=[]  NOutMax=[]  SumOutMin=[]  SumOutMax=[]  SaturationOutMin=[]  SaturationOutMax=[]  PParamMin=[]  PParamMax=[]  IParamMin=[]  IParamMax=[]  DParamMin=[]  DParamMax=[]  NParamMin=[]  NParamMax=[]  KbParamMin=[]  KbParamMax=[]  KtParamMin=[]  KtParamMax=[]  KbOutMin=[]  KbOutMax=[]  KtOutMin=[]  KtOutMax=[]  IntegratorOutMin=[]  IntegratorOutMax=[]  FilterOutMin=[]  FilterOutMax=[]  SumI1OutMin=[]  SumI1OutMax=[]  SumI2OutMin=[]  SumI2OutMax=[]  SumI3OutMin=[]  SumI3OutMax=[]  SumI4OutMin=[]  SumI4OutMax=[]  SumDOutMin=[]  SumDOutMax=[]  DifferentiatorOutMin=[]  DifferentiatorOutMax=[]  FilterDiffOutCoefMin=[]  FilterDiffOutCoefMax=[]  ReciprocalOutMin=[]  ReciprocalOutMax=[]  SumDenOutMin=[]  SumDenOutMax=[]  SumNumOutMin=[]  SumNumOutMax=[]  DivideOutMin=[]  DivideOutMax=[]  UdiffTsProdOutMin=[]  UdiffTsProdOutMax=[]  NTsProdOutMin=[]  NTsProdOutMax=[]  UintegralTsProdOutMin=[]  UintegralTsProdOutMax=[]  UngainTsProdOutMin=[]  UngainTsProdOutMax=[]  ClampingZeroOutDataTypeStr=Inherit: Inherit via back propagation  ClampingZeroOutMin=[]  ClampingZeroOutMax=[]  FilterDenConstantOutDataTypeStr=Inherit: Inherit via back propagation  FilterDenConstantOutMin=[]  FilterDenConstantOutMax=[]  PCopyOutDataTypeStr=Inherit: Inherit via back propagation  PCopyOutMin=[]  PCopyOutMax=[]  NCopyOutDataTypeStr=Inherit: Inherit via back propagation  NCopyOutMin=[]  NCopyOutMax=[]  IntegratorContinuousStateAttributes=''  IntegratorStateMustResolveToSignalObject=off  IntegratorRTWStateStorageClass=Auto  FilterContinuousStateAttributes=''  FilterStateMustResolveToSignalObject=off  FilterRTWStateStorageClass=Auto  ParallelPVariant=InternalParameters  IdealPVariant=Disabled  IVariant=InternalParameters  DVariant=InternalParameters  IntegratorVariant=Continuous  SatVariant=Enabled  AWVariant=BackCalculation  PCopyVariant=Disabled  TRVariant=Disabled  FdbkBlocksVariant=Forward  IdealPFdbkVariant=Disabled  SatFdbkVariant=Disabled  DerivativeFilterVariant=ContFilter  NVariant=InternalParameters  NCopyVariant=Disabled  FilterICVariant=InternalICsFilter  IntegratorICVariant=InternalICs  ExternalResetVariant=Disabled  TRSumVariant=Passthrough  SumFdbkVariant=Disabled  SumVariant=Sum_PID  TsampFilterVariant=InternalTs  TsampNgainVariant=Passthrough  TsampIntegralVariant=Passthrough  ExternalSaturationOutDataTypeStr=Inherit: Same as second input
  Product : Product  Inputs=3
  Product1 : Product
  Selector : Selector  InputPortWidth=4  IndexOptions=Index vector (dialog)  Indices=2  OutputSizes=1
  Sum : Sum  Inputs=|+-
  Terminator : Terminator
  w_cmp [rad/s] : Outport
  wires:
  F0003_reactionFlow.m/2 -> Selector/1
  Oxygen stoichiometry reference/1 -> Product/1
  Selector/1 -> Gain1/1
  Oxygen mass fraction in dry air/1 -> Product1/2
  F0003_reactionFlow.m/1 -> Terminator/1
  Gain1/1 -> Product/3
  Cells in FC stack/1 -> Product/2
  Product/1 -> Sum/1
  Product1/1 -> Sum/2
  Sum/1 -> Gain/1
  PID Controller/1 -> w_cmp [rad/s]/1
  Gain/1 -> PID Controller/1
  I_fc [A]/1 -> F0003_reactionFlow.m/1
  W_ca [kg/s]/1 -> Product1/1

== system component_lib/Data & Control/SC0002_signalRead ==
  SigIdentifier : Inport
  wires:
  SigIdentifier/1 -> [SigIdentifier]

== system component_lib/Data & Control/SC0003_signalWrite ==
  y : Outport
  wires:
  [SigIdentifier] -> y/1

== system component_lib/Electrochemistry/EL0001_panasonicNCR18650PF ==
  note: Kelvin -> degC
  I [A] : Inport
  T [K] : Inport  Port=2
  Abs : Abs
  Constant : Constant  Value=273.15
  Constant5 : Constant  Value=3.6e3
  Divide1 : Product  Inputs=*//
  F0001_cellCapacity.m : base_lib/F0001_panasonicCell/F0001_cellCapacity.m  SystemSampleTime=-1  VariantActivationTime=update diagram  Latency=0  AutoFrameSizeCalculation=off
  F0001_dynamicVoltage.m : base_lib/F0001_panasonicCell/F0001_dynamicVoltage.m  SystemSampleTime=-1  VariantActivationTime=update diagram  Latency=0  AutoFrameSizeCalculation=off
  F0001_ocvSOC.m : base_lib/F0001_panasonicCell/F0001_ocvSOC.m  SystemSampleTime=-1  VariantActivationTime=update diagram  Latency=0  AutoFrameSizeCalculation=off
  Gain : Gain  Gain=-1
  Integrator Limited : Integrator  InitialCondition=par.init_SOC  LimitOutput=on  UpperSaturationLimit=1  LowerSaturationLimit=0
  Integrator1 : Integrator  InitialCondition=zeros(5,1)
  Product : Product
  Saturation : Saturate  UpperLimit=0.9  LowerLimit=0.1
  Sum : Sum  Inputs=|+-
  Sum2 : Sum  Inputs=|+-
  V [V] : Outport
  SOC [-] : Outport  Port=2
  Q_gen [J/s] : Outport  Port=3
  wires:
  F0001_dynamicVoltage.m/1 -> Integrator1/1
  Integrator1/1 -> F0001_dynamicVoltage.m/1
  T [K]/1 -> Sum2/1
  F0001_ocvSOC.m/1 -> Sum/1
  Integrator Limited/1 -> SOC [-]/1, Saturation/1
  Constant/1 -> Sum2/2
  Sum2/1 -> F0001_dynamicVoltage.m/2, F0001_cellCapacity.m/1
  Constant5/1 -> Divide1/2
  F0001_cellCapacity.m/1 -> Divide1/3
  Gain/1 -> Divide1/1
  Divide1/1 -> Integrator Limited/1
  Saturation/1 -> F0001_ocvSOC.m/1
  F0001_dynamicVoltage.m/2 -> Product/1, Sum/2
  Sum/1 -> V [V]/1
  Abs/1 -> Q_gen [J/s]/1
  Product/1 -> Abs/1
  I [A]/1 -> F0001_dynamicVoltage.m/3, Gain/1, Product/2

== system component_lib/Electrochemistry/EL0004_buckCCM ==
  V_in [V] : Inport
  I_out [A] : Inport  Port=2
  d [-] : Inport  Port=3
  Abs : Abs
  Gain2 : Gain  Gain=1/C
  Gain4 : Gain  Gain=1/L
  Gain6 : Gain  Gain=R
  Integrator : Integrator
  Product{,1..3} (4 alike) : Product
  Saturation1 : Saturate  UpperLimit=1  LowerLimit=0
  Sum : Sum  Inputs=+|-
  Sum1 : Sum  Inputs=-+|
  Sum3 : Sum  Inputs=+-|
  Sum4 : Sum  Inputs=|++
  Transfer Fcn : TransferFcn  Denominator=[0.001 1]
  V_4 : Integrator  InitialCondition=V_init
  V_out [V] : Outport
  I_in [A] : Outport  Port=2
  Q_gen [J/s] : Outport  Port=3
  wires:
  Abs/1 -> Q_gen [J/s]/1
  Gain4/1 -> Integrator/1
  Gain6/1 -> Sum4/2
  Sum4/1 -> Sum1/1
  Sum1/1 -> Gain4/1
  Gain2/1 -> V_4/1
  Sum3/1 -> Gain2/1
  I_out [A]/1 -> [I_out], Sum3/2
  d [-]/1 -> Saturation1/1
  Integrator/1 -> Product/1, Gain6/1, Sum3/1
  Product1/1 -> Sum1/2
  Saturation1/1 -> Product1/2, Product/2
  Product/1 -> Transfer Fcn/1
  [I_out] -> Product2/2
  Sum/1 -> Abs/1
  V_in [V]/1 -> Product3/2, Product1/1
  Product3/1 -> Sum/2
  Product2/1 -> Sum/1
  V_4/1 -> Product2/1, V_out [V]/1, Sum4/1
  Transfer Fcn/1 -> Product3/1, I_in [A]/1

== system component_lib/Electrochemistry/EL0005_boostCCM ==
  note: Efficiency
  V_in [V] : Inport
  d [-] : Inport  Port=2
  I_out [A] : Inport  Port=3
  Abs : Abs
  Add : Sum  Inputs=+-
  Add1 : Sum  Inputs=+-
  Add2 : Sum  Inputs=+--
  Capacitor voltage : Integrator  InitialCondition=V_init
  Constant : Constant
  Constant1 : Constant  Value=eta
  Divide1 : Product  Inputs=**
  Gain : Gain  Gain=1/L
  Gain1 : Gain  Gain=1/C
  Gain2 : Gain  Gain=-1
  Integrator : Integrator
  Power : Math  Operator=pow
  Product{,1..3} (4 alike) : Product
  Resistor to ground : Gain  Gain=1e-4
  Saturation : Saturate  UpperLimit=0.8  LowerLimit=0.2
  Sign : Signum
  Sum : Sum  Inputs=+|-
  Transfer Fcn : TransferFcn  Denominator=[0.001 1]
  V_out [V] : Outport
  I_in [A] : Outport  Port=2
  Q_gen [J/s] : Outport  Port=3
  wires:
  Divide1/1 -> I_in [A]/1, [I_in], Gain2/1
  Abs/1 -> Q_gen [J/s]/1
  Sum/1 -> Abs/1
  [V_out] -> Product2/1
  [V_in] -> Product3/1
  [I_out] -> Product2/2
  [I_in] -> Product3/2
  Product2/1 -> Sum/1
  Product3/1 -> Sum/2
  Power/1 -> Divide1/2
  Transfer Fcn/1 -> Sign/1
  Gain2/1 -> Transfer Fcn/1
  Sign/1 -> Power/2
  Constant1/1 -> Power/1
  Resistor to ground/1 -> Add2/3
  V_in [V]/1 -> Add1/1, [V_in]
  d [-]/1 -> Saturation/1
  I_out [A]/1 -> Add2/2, [I_out]
  Gain1/1 -> Capacitor voltage/1
  Add2/1 -> Gain1/1
  Product1/1 -> Add2/1
  Integrator/1 -> Product1/1, Divide1/1
  Add1/1 -> Gain/1
  Product/1 -> Add1/2
  Add/1 -> Product1/2, Product/1
  Gain/1 -> Integrator/1
  Capacitor voltage/1 -> V_out [V]/1, [V_out], Product/2, Resistor to ground/1
  Constant/1 -> Add/1
  Saturation/1 -> Add/2

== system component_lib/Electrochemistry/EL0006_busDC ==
  V_1 [V] : Inport
  I_load [A] : Inport  Port=2
  V_2 [V] : Inport  Port=3
  Gain : Gain  Gain=1/C
  Gain1 : Gain  Gain=1e-3
  Gain2 : Gain  Gain=1/L
  Gain3 : Gain  Gain=1/L
  Gain4 : Gain  Gain=R
  Gain6 : Gain  Gain=R
  Integrator : Integrator
  Integrator1 : Integrator
  Sum : Sum  Inputs=|+-
  Sum1 : Sum  Inputs=-+|
  Sum2 : Sum  Inputs=|+-
  Sum3 : Sum  Inputs=+-+
  Sum4 : Sum  Inputs=|++
  Sum5 : Sum  Inputs=++|
  V_4 : Integrator  InitialCondition=V_init
  I_1 [A] : Outport
  V_bus [V] : Outport  Port=2
  I_2 [A] : Outport  Port=3
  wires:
  Gain1/1 -> Sum/2
  Sum/1 -> Gain/1
  Sum3/1 -> Sum/1
  V_4/1 -> V_bus [V]/1, Sum5/2, Gain1/1, Sum4/1
  I_load [A]/1 -> Sum3/2
  Gain/1 -> V_4/1
  Integrator/1 -> I_1 [A]/1, Gain4/1, Sum3/1
  Integrator1/1 -> I_2 [A]/1, Gain6/1, Sum3/3
  Sum1/1 -> Gain2/1
  V_1 [V]/1 -> Sum1/2
  Sum2/1 -> Gain3/1
  V_2 [V]/1 -> Sum2/1
  Gain2/1 -> Integrator/1
  Gain3/1 -> Integrator1/1
  Gain4/1 -> Sum4/2
  Sum4/1 -> Sum1/1
  Gain6/1 -> Sum5/1
  Sum5/1 -> Sum2/2
